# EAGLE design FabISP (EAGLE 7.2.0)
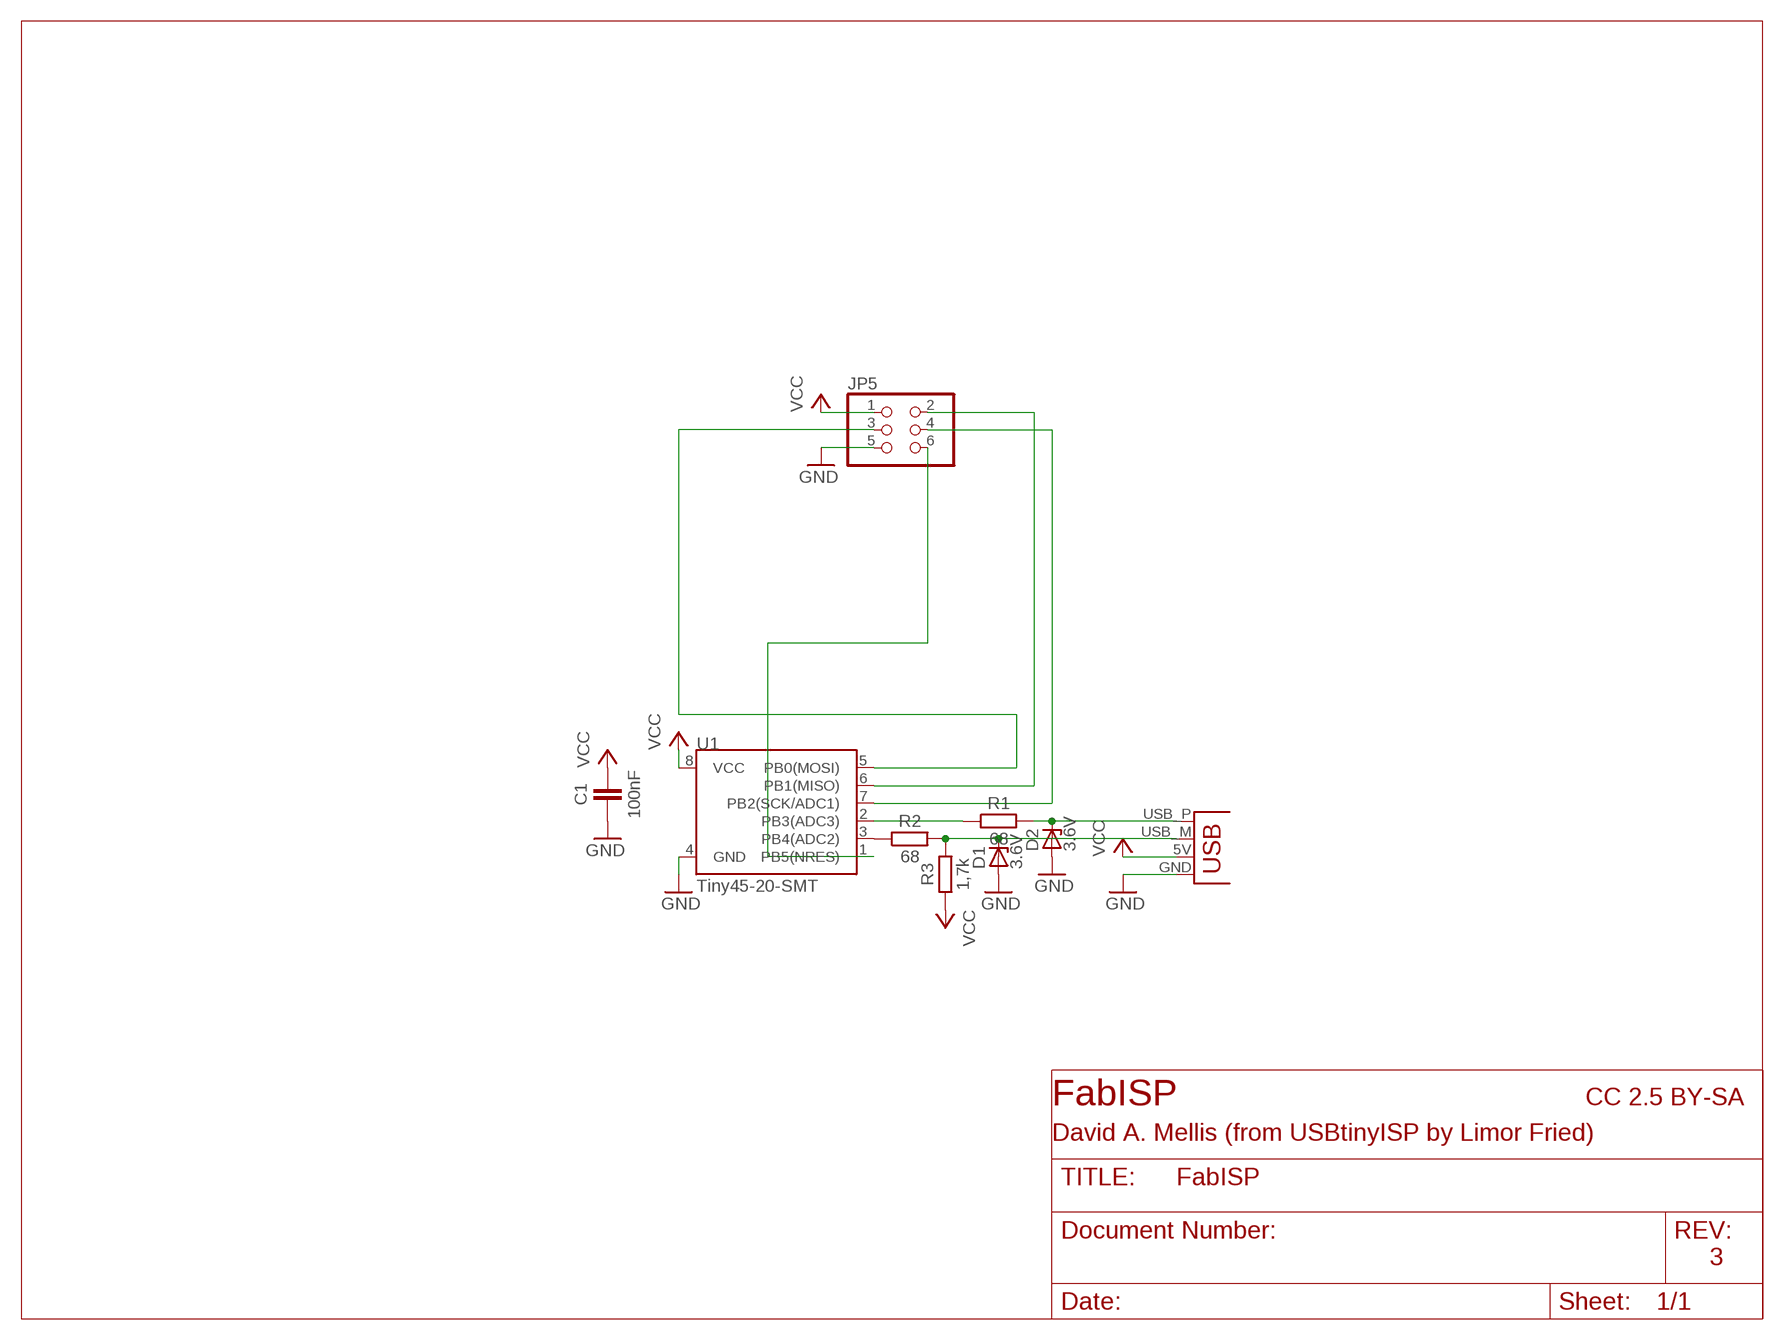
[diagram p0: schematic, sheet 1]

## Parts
C1  100nF  CAPACITOR1206  [1206]
D1  3.6V  ZENER_DIODESOD123  [SOD123]
D2  3.6V  ZENER_DIODESOD123  [SOD123]
JP4  USBPCB  [USB-A-PCB]
JP5  PINHD-2X3  [2X03]
R1  68  RESISTOR1206_WG  [1206_WIDEGAP]
R2  68  RESISTOR1206_WG  [1206_WIDEGAP]
R3  1,7k  RESISTOR1206_WG  [1206_WIDEGAP]
U1  Tiny45-20-SMT  ATTINY45TINY45-20-SMT  [SO08-EIAJ]

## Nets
GND: C1.1 D1.ANODE D2.ANODE JP4.GND JP5.5 U1.4(GND)
MISO: JP5.2 U1.6(PB1(MISO))
MOSI: JP5.3 U1.5(PB0(MOSI))
N$1: R1.1 U1.2(PB3(ADC3))
N$2: R2.1 U1.3(PB4(ADC2))
N$6: D1.CATHODE JP4.USB_M(D-) R2.2 R3.2
N$10: D2.CATHODE JP4.USB_P(D+) R1.2
RST: JP5.6 U1.1(PB5(NRES))
SCK: JP5.4 U1.7(PB2(SCK/ADC1))
VCC: C1.2 JP4.5V(VBUS) JP5.1 R3.1 U1.8(VCC)

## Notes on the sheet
- FabISP | CC 2.5 BY-SA
- David A. Mellis (from USBtinyISP by Limor Fried)
- 3

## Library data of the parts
C1 = thar:CAPACITOR
D1 D2 = ng:ZENER_DIODE: zener diode
JP4 = SparkFun-Connectors:USB: USB Connectors USB-B-PTH is fully proven SKU : PRT-00139/CONN-08278 USB-miniB is fully proven SKU : PRT-00587 USB-A-PCB is untested. USB-A-H is throughly reviewed, but untested. Spark Fun Electronics SKU : PRT-00437 USB-B-SMT is throughly reviewed, but untested. Needs silkscreen touching up.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
JP5 = pinhead:PINHD-2X3: PIN HEADER
R1-R3 = thar:RESISTOR
U1 = SparkFun-DigitalIC:ATTINY45: Atmel 8-pin 2/4/8kB flash uC; PROD_ID: IC-08922

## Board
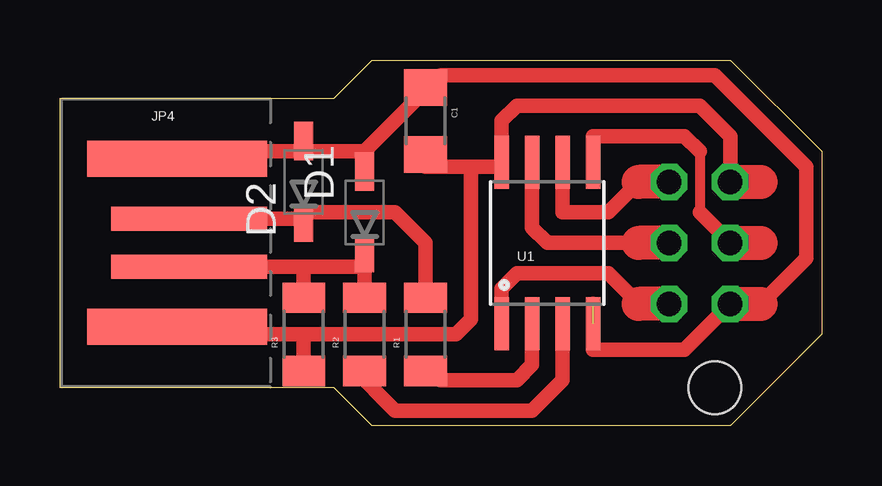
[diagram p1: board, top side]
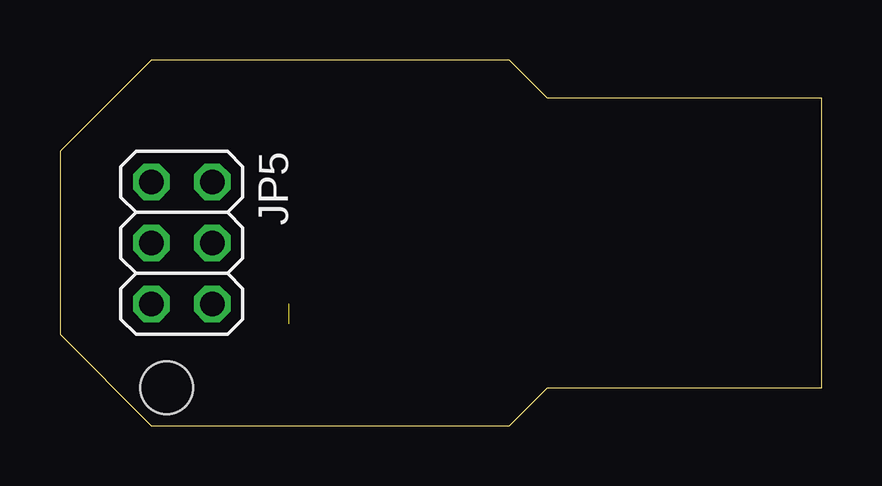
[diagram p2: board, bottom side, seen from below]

Size 31.75 x 15.24 mm. Coordinates in mm from the lower left corner, seen from the top.
Outline: 0,13.65 11.43,13.65 13.02,15.24 27.94,15.24 31.75,11.43 31.75,3.81 27.94,0 13.02,0 11.43,1.59 0,1.59 0,13.65
Copper layers (1*16): Top 0.035mm / dielectric 1.5mm / Bottom 0.035mm
Design rules "default *": minimum track width 12mil, minimum drill 24mil, track to track 17mil, track to pad 16mil, pad to pad 16mil, via to via 16mil, smd to smd 0mil, copper to edge 17mil, drill to drill 8mil, minimum pad ring 10mil, minimum via ring 8mil, stop-mask expansion 4mil, vias tented up to drill 0mil, thermal gap 10mil
Holes 2.2 mm at 27.3,1.59

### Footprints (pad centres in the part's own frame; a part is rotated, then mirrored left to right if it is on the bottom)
1206 = smd 1.524 x 1.778: 1 -1.397,0; 2 1.397,0
SOD123 = smd 1.6 x 0.8: ANODE 1.7,0; CATHODE -1.7,0
USB-A-PCB = smd 7.5 x 1.5: 5V -0.2,-3.5; GND -0.2,3.5 | smd 6.5 x 1: USB_M 0.3,-1; USB_P 0.3,1
2X03 = drill 1.016 octagon: 1 -2.54,-1.27; 2 -2.54,1.27; 3 0,-1.27; 4 0,1.27; 5 2.54,-1.27; 6 2.54,1.27
1206_WIDEGAP = smd 1.27 x 1.778: 1 -1.524,0; 2 1.524,0
SO08-EIAJ = smd 0.61 x 2.21: 1 -1.905,-3.378; 2 -0.635,-3.378; 3 0.635,-3.378; 4 1.905,-3.378; 5 1.905,3.353; 6 0.635,3.353; 7 -0.635,3.353; 8 -1.905,3.353

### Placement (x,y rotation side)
C1  15.24,12.7 270 top
D1  12.7,8.89 90 top
D2  10.16,10.16 90 top
JP4  5.08,7.62 0 top
JP5  26.67,7.62 270 bottom
R1  15.24,3.81 90 top
R2  12.7,3.81 90 top
R3  10.16,3.81 90 top
U1  20.32,7.62 0 top

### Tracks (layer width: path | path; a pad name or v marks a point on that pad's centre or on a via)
GND  (1 unrouted)
  Top 0.61: 22.23,5.08 22.23,3.17 26.04,3.17 JP5.5 | JP4.GND 6.04,11.12 6.35,11.43 10.16,11.43 | 10.16,11.43 12.7,11.43 | D1.ANODE 12.7,11.43 | D2.ANODE 10.16,11.43 | 12.7,11.43 15.24,13.97 | 15.24,13.97 15.87,14.6 27.3,14.6 31.11,10.79 31.11,6.99 29.21,5.08 | C1.1 15.24,13.97
  Top 1.422: JP5.5 29.21,5.08
MISO
  Top 0.61: U1.6 20.96,8.89 22.86,8.89 24.13,10.16
  Top 1.422: JP5.2 24.13,10.16
MOSI
  Top 0.406: 26.67,11.43 26.67,8.89
  Top 0.61: JP5.3 26.67,8.89 | 26.67,11.43 26.04,12.06 22.23,12.06 U1.5
  Top 1.422: JP5.3 29.21,7.62
N$1
  Top 0.61: U1.2 19.69,2.54 19.05,1.9 15.87,1.9 15.24,2.54 R1.1
N$2
  Top 0.61: U1.3 20.96,1.9 19.69,0.63 13.97,0.63 12.19,2.41 R2.1
N$6
  Top 0.61: JP4.USB_M 10.16,6.62 | 10.16,6.62 12.7,6.62 D1.CATHODE R2.2 | R3.2 10.16,6.62
N$10
  Top 0.61: JP4.USB_P 10.16,8.62 | D2.CATHODE 10.16,8.62 | 10.16,8.62 10.16,8.89 13.97,8.89 15.24,7.62 R1.2
RST
  Top 0.61: U1.1 18.42,5.71 19.05,6.35 22.86,6.35 24.13,5.08
  Top 1.422: JP5.6 24.13,5.08
SCK
  Top 0.61: U1.7 19.69,8.26 20.32,7.62 24.13,7.62
  Top 1.422: JP5.4 24.13,7.62
VCC
  Top 0.61: JP5.1 27.94,12.06 26.67,13.33 19.05,13.33 18.42,12.7 U1.8 18.24,10.79 17.14,10.79 | JP4.5V 4.88,4.01 5.08,3.81 10.16,3.81 | 10.16,3.81 16.51,3.81 17.14,4.45 17.14,10.79 | R3.1 10.16,3.81 | C1.2 15.24,10.79 17.14,10.79
  Top 1.422: JP5.1 29.21,10.16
